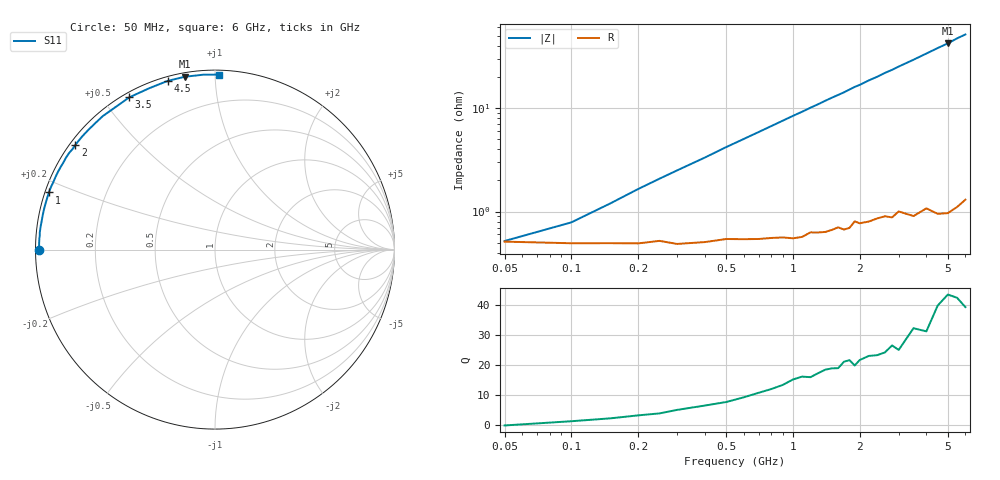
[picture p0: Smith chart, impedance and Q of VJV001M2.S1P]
! Infineon Technologies  Discrete & RF Semiconductors
! BB 914
! Si Tuning Diode in SOT23
! VR =
! S-Parameters:  July  1999
# GHz  S  MA  R  50
!  f  S11
! GHz  MAG  ANG
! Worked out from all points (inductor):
!   34 points, 50 MHz to 6 GHz, reference 50 ohm
!   read as one part to ground: L = 1.28 nH near 200 MHz
!   highest Q = 42.5 at 5 GHz (marker M1), where L = 1.34 nH
!   S11 on the Smith chart (normalised r, x): 50 MHz: 0.01, -0.00; 1 GHz: 0.01, +0.17; 2 GHz: 0.02, +0.33; 3.5 GHz: 0.02, +0.58; 4.5 GHz: 0.02, +0.76; 6 GHz: 0.03, +1.02
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0.05  0.9797 -179.8
0.1  0.9805 178.6
0.2  0.9805 176.4
0.25  0.9794 175.4
0.3  0.9808 174.4
0.4  0.98 172.5
0.6  0.9788 168.6
0.8  0.9784 164.8
1  0.9788 161.0
1.1  0.9782 159.2
1.4  0.9762 153.6
1.5  0.9753 151.8
1.6  0.9741 150.1
1.7  0.9755 148.4
1.8  0.9748 146.5
1.9  0.9713 144.6
2  0.9727 143.1
2.2  0.9722 139.5
2.4  0.9709 136.4
2.6  0.9702 132.9
2.8  0.9716 130.0
3  0.9685 126.7
3.5  0.9734 119.4
4  0.9708 112.3
4.5  0.9762 105.7
5  0.9776 99.9
5.5  0.9768 93.6
6  0.9749 88.6
